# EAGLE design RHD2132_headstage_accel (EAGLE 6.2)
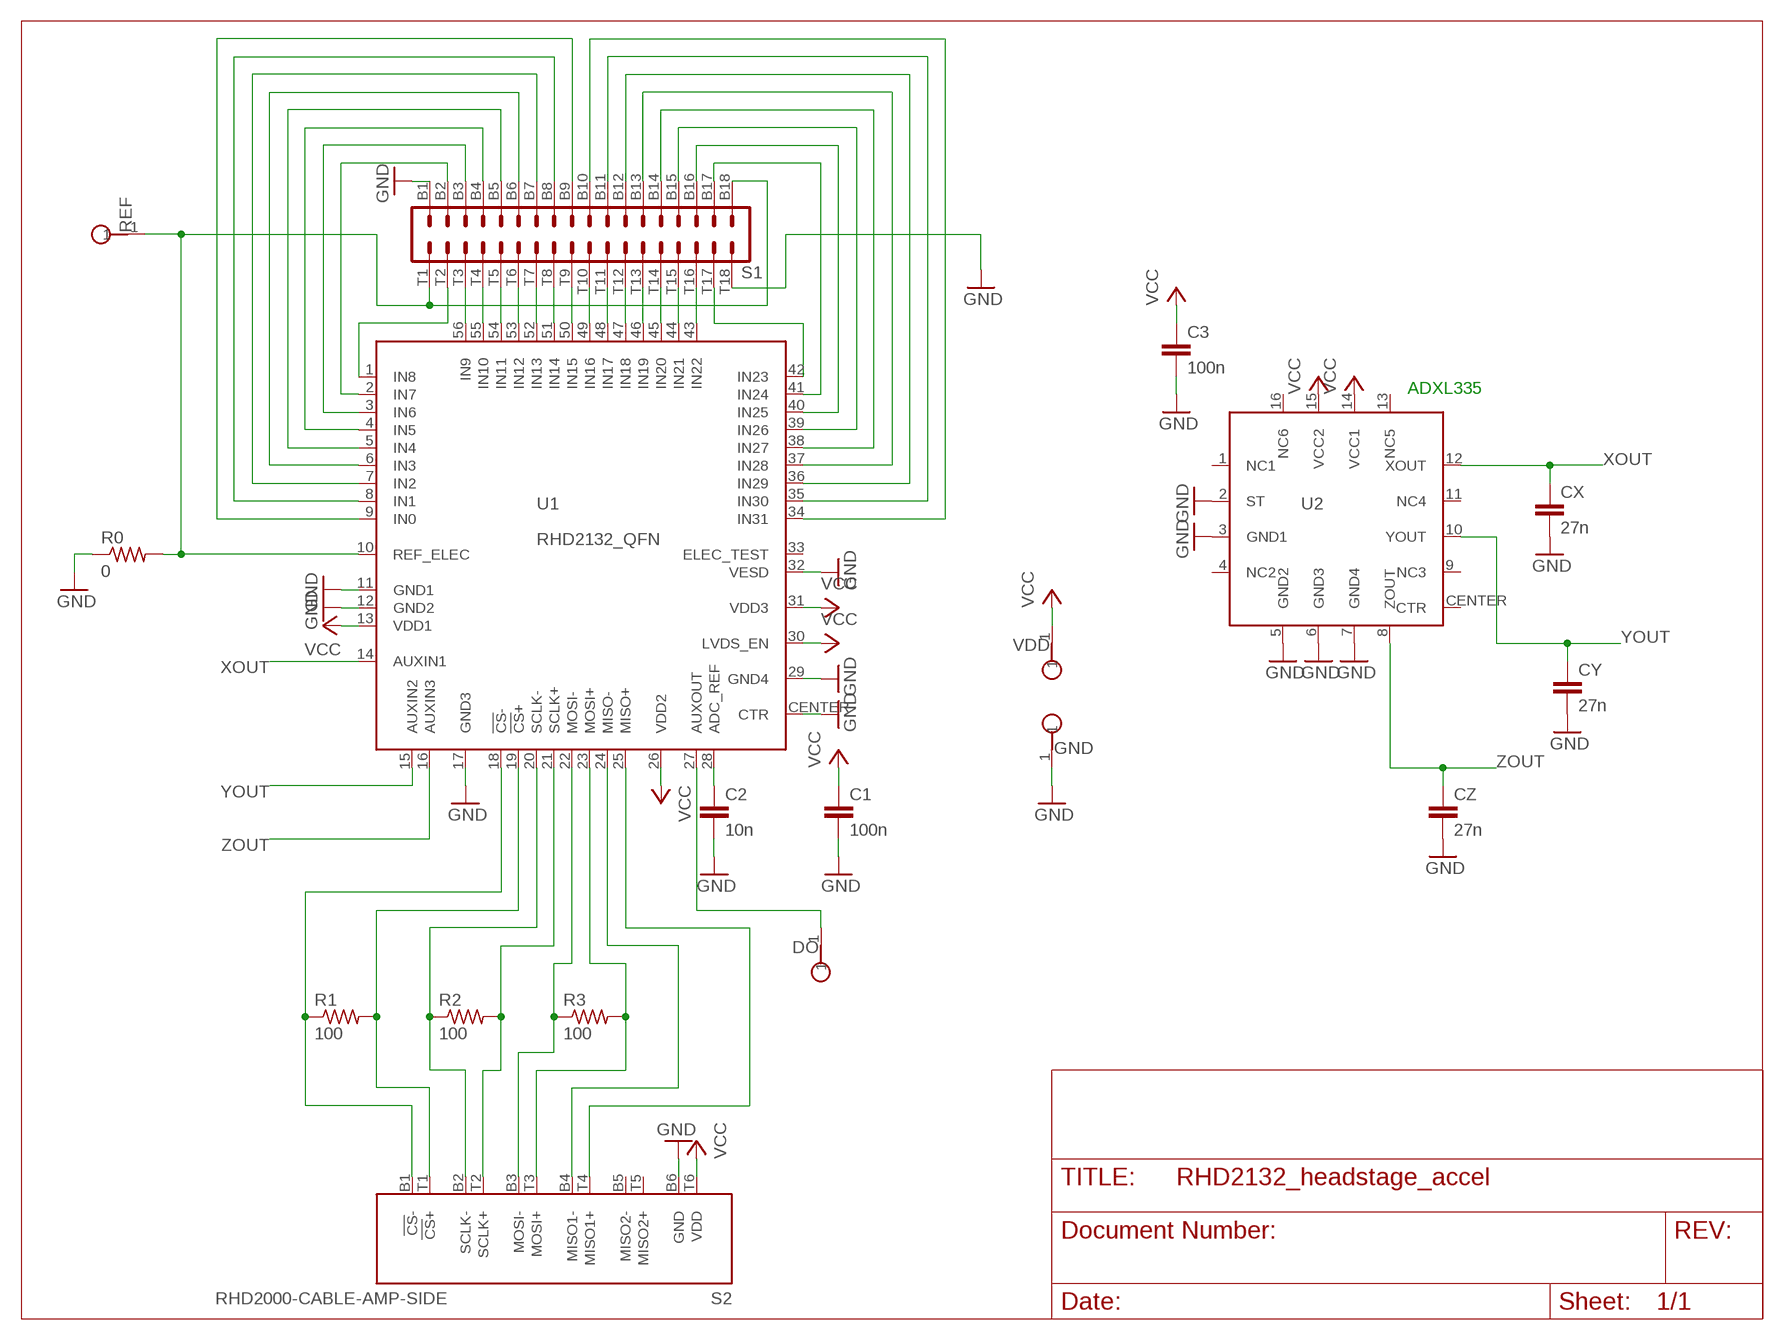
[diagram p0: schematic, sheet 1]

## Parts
C1  100n  C_0402  [0402]
C2  10n  C_0402  [0402]
C3  100n  C_0402  [0402]
CX  27n  C_0402  [0402]
CY  27n  C_0402  [0402]
CZ  27n  C_0402  [0402]
DO  TESTPOINT_SMALL  [TESTPOINT_SMALL]
GND  TESTPOINT_SMALL  [TESTPOINT_SMALL]
R0  0  R_0402  [0402]
R1  100  R_0402  [0402]
R2  100  R_0402  [0402]
R3  100  R_0402  [0402]
REF  TESTPOINT_SMALL  [TESTPOINT_SMALL]
S1  OMNETICS_A79025  [OMNETICS_A79025]
S2  RHD2000-CABLE-AMP-SIDE  [OMNETICS_PZN-12-AA]
U1  RHD2132_QFN  [QFN56_8_X_8_LARGE]
U2  ADXL335  [ADXL335]
VDD  TESTPOINT_SMALL  [TESTPOINT_SMALL]

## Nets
GND: C1.2 C2.2 C3.2 CX.2 CY.2 CZ.2 GND.1 R0.1 S1.B1 S1.T18 S2.B6(GND) U1.11(GND1) U1.12(GND2) U1.17(GND3) U1.29(GND4) U1.32(VESD) U1.CENTER(CTR) U2.2(ST) U2.3(GND1) U2.5(GND2) U2.6(GND3) U2.7(GND4)
N$1: R0.2 REF.1 S1.B18 S1.T1 U1.10(REF_ELEC)
N$2: S1.B3 U1.3(IN6)
N$3: S1.B2 U1.2(IN7)
N$4: S1.B4 U1.4(IN5)
N$5: S1.B5 U1.5(IN4)
N$6: S1.B6 U1.6(IN3)
N$7: S1.B7 U1.7(IN2)
N$8: S1.B8 U1.8(IN1)
N$9: S1.B9 U1.9(IN0)
N$10: S1.B10 U1.34(IN31)
N$11: R1.1 S2.B1(!CS!-) U1.18(!CS!-)
N$12: S1.B17 U1.41(IN24)
N$13: S1.B16 U1.40(IN25)
N$14: S1.B15 U1.39(IN26)
N$15: S1.B14 U1.38(IN27)
N$16: S1.B13 U1.37(IN28)
N$17: S1.B12 U1.36(IN29)
N$18: S1.B11 U1.35(IN30)
N$19: S1.T9 U1.50(IN15)
N$20: S1.T8 U1.51(IN14)
N$21: S1.T7 U1.52(IN13)
N$22: S1.T3 U1.56(IN9)
N$23: S1.T4 U1.55(IN10)
N$24: S1.T5 U1.54(IN11)
N$25: S1.T6 U1.53(IN12)
N$26: S1.T10 U1.49(IN16)
N$27: S1.T11 U1.48(IN17)
N$28: S1.T12 U1.47(IN18)
N$29: S1.T13 U1.46(IN19)
N$30: S1.T14 U1.45(IN20)
N$31: S1.T15 U1.44(IN21)
N$32: S1.T16 U1.43(IN22)
N$33: S1.T2 U1.1(IN8)
N$34: S1.T17 U1.42(IN23)
N$35: R1.2 S2.T1(!CS!+) U1.19(!CS!+)
N$36: R2.1 S2.B2(SCLK-) U1.20(SCLK-)
N$37: R2.2 S2.T2(SCLK+) U1.21(SCLK+)
N$38: R3.1 S2.B3(MOSI-) U1.22(MOSI-)
N$39: R3.2 S2.T3(MOSI+) U1.23(MOSI+)
N$40: S2.B4(MISO1-) U1.24(MISO-)
N$41: S2.T4(MISO1+) U1.25(MISO+)
N$42: C2.1 U1.28(ADC_REF)
N$43: DO.1 U1.27(AUXOUT)
VCC: C1.1 C3.1 S2.T6(VDD) U1.13(VDD1) U1.26(VDD2) U1.30(LVDS_EN) U1.31(VDD3) U2.14(VCC1) U2.15(VCC2) VDD.1
XOUT: CX.1 U1.14(AUXIN1) U2.12(XOUT)
YOUT: CY.1 U1.15(AUXIN2) U2.10(YOUT)
ZOUT: CZ.1 U1.16(AUXIN3) U2.8(ZOUT)
Unconnected: S2.B5(MISO2-) S2.T5(MISO2+) U1.33(ELEC_TEST) U2.1(NC1) U2.4(NC2) U2.9(NC3) U2.11(NC4) U2.13(NC5) U2.16(NC6) U2.CENTER(CTR)

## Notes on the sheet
- ADXL335

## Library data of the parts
C1-C3 CX CY CZ = RHD2000_eval_board:C: Capacitor
DO GND REF VDD = RHD2000_eval_board:TESTPOINT: PCB Test Point
R0 R1-R3 = RHD2000_eval_board:R: Resistor
S1 = RHD2000:OMNETICS_A79025
S2 = RHD2000:RHD2000-CABLE-AMP-SIDE
U1 = RHD2000:RHD2132
U2 = harrison:ADXL335

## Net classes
1 thick: width 1.016 mm
2 power: width 0.61 mm

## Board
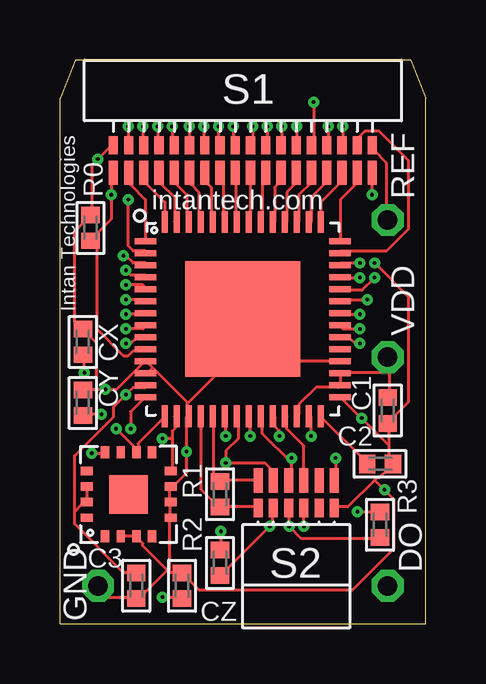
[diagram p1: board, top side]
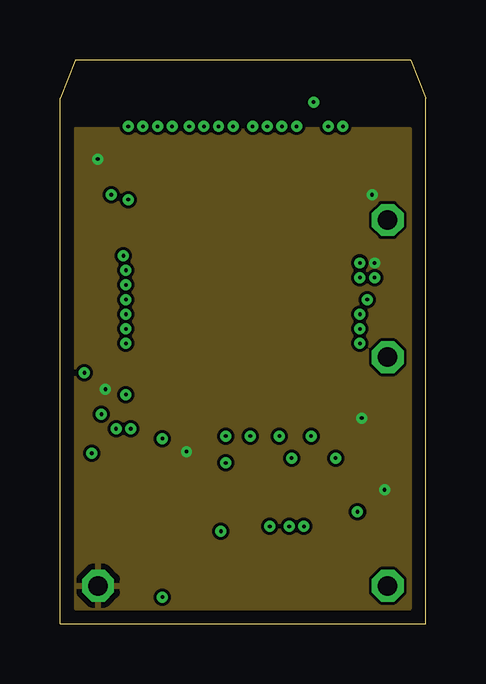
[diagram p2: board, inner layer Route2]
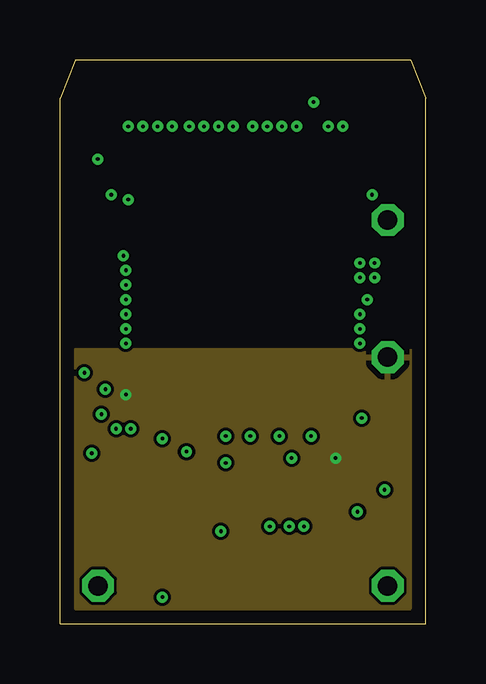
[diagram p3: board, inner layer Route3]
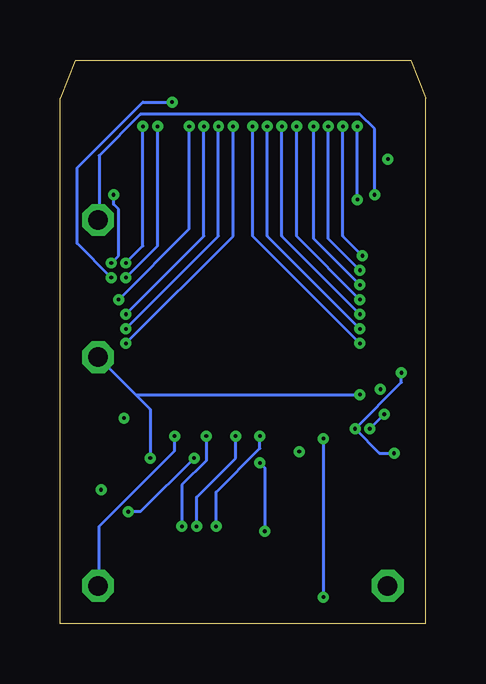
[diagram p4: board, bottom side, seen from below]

Size 15.24 x 23.5 mm. Coordinates in mm from the lower left corner, seen from the top.
Outline: 0,0 0,21.91 0.64,23.5 14.61,23.5 15.24,21.91 15.24,0 0,0
Copper layers (1*2+3*16): Top 0.035mm / dielectric 1.5mm / Route2 0.035mm / dielectric 0.15mm / Route3 0.035mm / dielectric 0.2mm / Bottom 0.035mm
Design rules: minimum track width 5mil, minimum drill 6mil, track to track 5mil, track to pad 5mil, pad to pad 5mil, via to via 5mil, smd to smd 5mil, copper to edge 15mil, drill to drill 15mil, minimum pad ring 10mil, minimum via ring 6mil, stop-mask expansion 4mil, vias tented up to drill 0mil, thermal gap 10mil

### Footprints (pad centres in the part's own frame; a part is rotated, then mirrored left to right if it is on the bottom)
0402 = smd 0.686 x 0.762: 1 -0.533,0; 2 0.533,0
TESTPOINT_SMALL = drill 0.813 octagon: 1 0,0
OMNETICS_A79025 = smd 0.381 x 0.762: B1 -5.397,-1.016; B2 -4.763,-1.016; B3 -4.128,-1.016; B4 -3.493,-1.016; B5 -2.857,-1.016; B6 -2.223,-1.016; B7 -1.587,-1.016; B8 -0.953,-1.016; B9 -0.318,-1.016; B10 0.318,-1.016; B11 0.953,-1.016; B12 1.587,-1.016; B13 2.223,-1.016; B14 2.857,-1.016; B15 3.493,-1.016; B16 4.128,-1.016; B17 4.763,-1.016; B18 5.397,-1.016 | smd 0.381 x 1.016: T1 -5.397,-2.159; T2 -4.763,-2.159; T3 -4.128,-2.159; T4 -3.493,-2.159; T5 -2.857,-2.159; T6 -2.223,-2.159; T7 -1.587,-2.159; T8 -0.953,-2.159; T9 -0.318,-2.159; T10 0.318,-2.159; T11 0.953,-2.159; T12 1.587,-2.159; T13 2.223,-2.159; T14 2.857,-2.159; T15 3.493,-2.159; T16 4.128,-2.159; T17 4.763,-2.159; T18 5.397,-2.159
OMNETICS_PZN-12-AA = smd 0.381 x 0.762: B1 1.587,-1.016; B2 0.953,-1.016; B3 0.318,-1.016; B4 -0.318,-1.016; B5 -0.953,-1.016; B6 -1.587,-1.016 | smd 0.381 x 1.016: T1 1.587,-2.159; T2 0.953,-2.159; T3 0.318,-2.159; T4 -0.318,-2.159; T5 -0.953,-2.159; T6 -1.587,-2.159
QFN56_8_X_8_LARGE = smd 0.9 x 0.25: 1 -4.05,3.25; 2 -4.05,2.75; 3 -4.05,2.25; 4 -4.05,1.75; 5 -4.05,1.25; 6 -4.05,0.75; 7 -4.05,0.25; 8 -4.05,-0.25; 9 -4.05,-0.75; 10 -4.05,-1.25; 11 -4.05,-1.75; 12 -4.05,-2.25; 13 -4.05,-2.75; 14 -4.05,-3.25; 29 4.05,-3.25; 30 4.05,-2.75; 31 4.05,-2.25; 32 4.05,-1.75; 33 4.05,-1.25; 34 4.05,-0.75; 35 4.05,-0.25; 36 4.05,0.25; 37 4.05,0.75; 38 4.05,1.25; 39 4.05,1.75; 40 4.05,2.25; 41 4.05,2.75; 42 4.05,3.25 | smd 0.25 x 0.9: 15 -3.25,-4.05; 16 -2.75,-4.05; 17 -2.25,-4.05; 18 -1.75,-4.05; 19 -1.25,-4.05; 20 -0.75,-4.05; 21 -0.25,-4.05; 22 0.25,-4.05; 23 0.75,-4.05; 24 1.25,-4.05; 25 1.75,-4.05; 26 2.25,-4.05; 27 2.75,-4.05; 28 3.25,-4.05; 43 3.25,4.05; 44 2.75,4.05; 45 2.25,4.05; 46 1.75,4.05; 47 1.25,4.05; 48 0.75,4.05; 49 0.25,4.05; 50 -0.25,4.05; 51 -0.75,4.05; 52 -1.25,4.05; 53 -1.75,4.05; 54 -2.25,4.05; 55 -2.75,4.05; 56 -3.25,4.05 | smd 4.8 x 4.8: CENTER 0,0
ADXL335 = smd 0.5 x 0.35: 1 -1.75,0.975; 2 -1.75,0.325; 3 -1.75,-0.325; 4 -1.75,-0.975; 9 1.75,-0.975; 10 1.75,-0.325; 11 1.75,0.325; 12 1.75,0.975 | smd 0.35 x 0.5: 5 -0.975,-1.75; 6 -0.325,-1.75; 7 0.325,-1.75; 8 0.975,-1.75; 13 0.975,1.75; 14 0.325,1.75; 15 -0.325,1.75; 16 -0.975,1.75 | smd 1.6 x 1.6: CENTER 0,0

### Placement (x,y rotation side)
C1  13.65,8.89 270 top
C2  13.34,6.67 0 top
C3  3.17,1.59 270 top
CX  0.95,11.75 90 top
CY  0.95,9.21 90 top
CZ  5.08,1.59 90 top
DO  13.65,1.59 0 top
GND  1.59,1.59 0 top
R0  1.27,16.5 270 top
R1  6.67,5.4 90 top
R2  6.67,2.54 90 top
R3  13.34,4.13 90 top
REF  13.65,16.83 90 top
S1  7.62,20.95 0 top
S2  9.84,3.81 180 top
U1  7.62,12.7 0 top
U2  2.86,5.4 90 top
VDD  13.65,11.11 0 top

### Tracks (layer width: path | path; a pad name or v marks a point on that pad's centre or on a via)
GND  (via drill 0.15)
  Top 0.127: 8.23,12.09 9.35,10.97 11.58,10.97 U1.32 | S1.B1 2.13,19.91 1.32,19.1 1.32,17.07 R0.1 1.22,16.97 0.61,16.36 0.61,12.6 0.91,12.29 CX.2 1.02,12.19 1.52,11.68 1.52,9.75 | 1.52,9.75 2.34,9.75 3.56,10.97 U1.11 3.66,10.87 3.86,10.67 | 1.52,9.75 1.02,9.75 CY.2 | 5.28,9.14 5.28,9.25 3.86,10.67 | 5.28,9.14 5.28,8.74 U1.17 5.28,8.64 5.28,6.3 4.67,5.69 U2.7 4.57,5.69 4.57,5.08 U2.6 4.57,4.98 4.57,4.47 U2.5 4.57,4.37 4.57,2.13 | 3.86,10.67 3.66,10.46 U1.12 | 5.28,9.14 8.23,12.09 | 8.23,12.09 U1.CENTER | 13.11,5.99 13.21,6.1 13.31,6.1 13.72,6.5 | 13.11,5.99 11.99,4.88 11.48,4.88 S2.B6 | 13.72,6.5 13.82,6.6 C2.2 13.72,6.5 | 13.72,6.5 13.72,7.42 | 13.72,7.42 13.72,8.33 C1.2 13.72,8.43 14.53,9.25 14.53,13.61 v13.11,15.04 | 13.72,7.42 11.68,9.45 U1.29 | U2.2 3.15,3.66 U2.3 3.25,3.56 3.45,3.35 3.45,3.25 4.47,2.23 | 4.57,2.13 4.47,2.23 | 5.08,2.13 4.57,2.13 | GND.1 1.63,1.52 2.03,1.12 3.15,1.12 C3.2 3.25,1.02 4.47,2.23 | 13.11,5.99 13.92,5.18 13.92,3.15 12.19,1.42 5.79,1.42 5.08,2.13 | 5.08,2.13 CZ.2 | v13.01,17.88 13.01,18.8 S1.T18
  Bottom 0.127: v13.01,17.88 13.01,17.48 12.8,17.27 12.8,15.34 v13.11,15.04
  other vias: 12.57,8.57 13.53,5.59 5.27,7.18 1.57,19.37 1.89,9.78
  pour Route2: 0.64,0.64 14.61,0.64 14.61,20.64 0.64,20.64
N$1  (via drill 0.15)
  Top 0.127: S1.B18 13.11,19.91 13.11,19.71 13.61,19.2 13.61,16.87 REF.1 | 1.52,16.26 2.13,16.87 v2.13,17.88 2.13,18.8 S1.T1 | 1.52,16.26 1.32,16.05 R0.2 1.52,16.26 | 1.52,16.26 1.52,12.29 2.64,11.18 2.85,11.18 3.05,11.38 3.56,11.38 U1.10
  Bottom 0.127: v2.13,17.88 2.13,20.62 2.74,21.23 11.89,21.23 13.61,19.51 13.61,16.87 REF.1
N$2  (via drill 0.15)
  Top 0.127: v3.45,20.73 3.45,20.02 S1.B3 | v2.64,15.34 2.74,15.34 3.05,15.04 3.56,15.04 U1.3
  Bottom 0.127: v3.45,20.73 3.45,16.15 v2.64,15.34
N$3  (via drill 0.15)
  Top 0.127: v2.85,20.73 2.85,20.02 S1.B2 | v2.85,17.68 2.85,15.75 3.05,15.54 3.56,15.54 U1.2
  Bottom 0.127: v2.85,17.68 v2.85,20.73
N$4  (via drill 0.15)
  Top 0.127: v4.06,20.73 4.06,20.02 S1.B4 | v2.74,14.73 2.95,14.53 3.56,14.53 U1.4
  Bottom 0.127: v4.06,20.73 4.06,16.05 v2.74,14.73
N$5  (via drill 0.15)
  Top 0.127: v4.67,20.73 4.67,20.02 S1.B5 | v2.74,14.12 3.45,14.12 3.56,14.02 U1.5
  Bottom 0.127: v4.67,20.73 4.67,16.05 v2.74,14.12
N$6  (via drill 0.15)
  Top 0.127: v5.38,20.73 5.38,20.02 S1.B6 | v2.74,13.51 3.56,13.51 U1.6
  Bottom 0.127: v5.38,20.73 5.38,16.15 v2.74,13.51
N$7  (via drill 0.15)
  Top 0.127: v5.99,20.73 5.99,20.02 S1.B7 | v2.74,12.9 3.56,12.9 U1.7
  Bottom 0.127: v5.99,20.73 5.99,16.15 v2.74,12.9
N$8  (via drill 0.15)
  Top 0.127: v6.6,20.73 6.6,20.02 S1.B8 | v2.74,12.29 3.45,12.29 3.56,12.39 U1.8
  Bottom 0.127: v6.6,20.73 6.6,16.15 v2.74,12.29
N$9  (via drill 0.15)
  Top 0.127: v7.21,20.73 7.21,20.02 S1.B9 | v2.74,11.68 2.95,11.68 3.15,11.89 3.56,11.89 U1.9
  Bottom 0.127: v7.21,20.73 7.21,16.15 v2.74,11.68
N$10  (via drill 0.15)
  Top 0.127: v8.03,20.73 8.03,20.02 S1.B10 | v12.5,11.68 12.29,11.68 12.09,11.89 11.68,11.89 U1.34
  Bottom 0.127: v8.03,20.73 8.03,16.15 v12.5,11.68
N$11
  Top 0.127: S2.B1 8.23,4.88 6.71,4.88 R1.1 6.6,4.88 5.89,5.59 5.89,8.64 U1.18
N$12
  Top 0.127: S1.B17 12.39,20.02 12.39,20.22 12.7,20.52 13.31,20.52 14.53,19.3 14.53,16.46 13.61,15.54 11.68,15.54 U1.41
N$13  (via drill 0.15)
  Top 0.127: v11.79,20.73 11.79,20.02 S1.B16 | v12.5,15.04 11.68,15.04 U1.40
  Bottom 0.127: v11.79,20.73 11.79,15.75 v12.5,15.04
N$14  (via drill 0.15)
  Top 0.127: v11.18,20.73 11.18,20.02 S1.B15 | v12.5,14.43 11.68,14.43 U1.39
  Bottom 0.127: v11.18,20.73 11.18,15.75 v12.5,14.43
N$15  (via drill 0.15)
  Top 0.127: v10.57,21.74 10.57,20.02 S1.B14 | v13.11,14.43 12.6,13.92 11.68,13.92 U1.38
  Bottom 0.127: v10.57,21.74 11.79,21.74 14.53,19 14.53,15.85 v13.11,14.43
N$16  (via drill 0.15)
  Top 0.127: v9.86,20.73 9.86,20.02 S1.B13 | v12.8,13.51 11.68,13.51 U1.37
  Bottom 0.127: v9.86,20.73 9.86,16.46 v12.8,13.51
N$17  (via drill 0.15)
  Top 0.127: v9.25,20.73 9.25,20.02 S1.B12 | v12.5,12.9 11.68,12.9 U1.36
  Bottom 0.127: v9.25,20.73 9.25,16.15 v12.5,12.9
N$18  (via drill 0.15)
  Top 0.127: v8.64,20.73 8.64,20.02 S1.B11 | v12.5,12.29 11.79,12.29 11.68,12.39 U1.35
  Bottom 0.127: v8.64,20.73 8.64,16.15 v12.5,12.29
N$19
  Top 0.127: U1.50 7.32,16.76 7.32,18.8 S1.T9
N$20
  Top 0.127: U1.51 6.81,16.76 6.81,18.69 6.71,18.8 S1.T8
N$21
  Top 0.127: U1.52 6.3,16.76 6.3,18.19 6.1,18.39 6.1,18.8 S1.T7
N$22
  Top 0.127: U1.56 4.37,16.76 4.37,17.58 3.56,18.39 3.56,18.8 S1.T3
N$23
  Top 0.127: U1.55 4.78,16.76 4.78,17.78 4.17,18.39 4.17,18.8 S1.T4
N$24
  Top 0.127: U1.54 5.28,16.76 5.28,17.88 4.78,18.39 4.78,18.8 S1.T5
N$25
  Top 0.127: U1.53 5.79,16.76 5.79,17.98 5.49,18.29 5.49,18.8 S1.T6
N$26
  Top 0.127: U1.49 7.92,16.76 7.92,18.8 S1.T10
N$27
  Top 0.127: U1.48 8.43,16.76 8.43,18.69 8.53,18.8 S1.T11
N$28
  Top 0.127: U1.47 8.94,16.76 8.94,18.19 9.14,18.39 9.14,18.8 S1.T12
N$29
  Top 0.127: U1.46 9.45,16.76 9.45,17.98 9.75,18.29 9.75,18.8 S1.T13
N$30
  Top 0.127: U1.45 9.96,16.76 9.96,17.88 10.46,18.39 10.46,18.8 S1.T14
N$31
  Top 0.127: U1.44 10.46,16.76 10.46,17.78 11.07,18.39 11.07,18.8 S1.T15
N$32
  Top 0.127: U1.43 10.87,16.76 10.87,17.58 11.68,18.39 11.68,18.8 S1.T16
N$33
  Top 0.127: U1.1 3.56,15.95 3.56,17.68 2.95,18.29 2.95,18.8 S1.T2
N$34
  Top 0.127: U1.42 11.68,15.95 11.68,17.68 12.29,18.29 12.29,18.8 S1.T17
N$35
  Top 0.127: S2.T1 8.23,5.99 6.71,5.99 R1.2 6.4,6.2 6.4,8.64 U1.19
N$36  (via drill 0.15)
  Top 0.127: R2.1 6.71,2.03 v8.74,4.06 8.84,4.17 8.84,4.78 S2.B2 | v6.91,7.82 6.91,8.64 U1.20
  Bottom 0.127: v6.91,7.82 6.91,7.32 8.74,5.49 v8.74,4.06
N$37  (via drill 0.15)
  Top 0.127: v6.71,3.86 6.71,3.15 R2.2 | U1.21 7.42,8.64 7.42,7.72 6.91,7.21 v6.91,6.71 8.53,6.71 8.84,6.4 8.84,5.99 S2.T2
  Bottom 0.127: v6.71,3.86 6.71,6.5 v6.91,6.71
N$38  (via drill 0.15)
  Top 0.127: S2.B3 9.55,4.78 v9.55,4.06 10.06,3.56 13.31,3.56 R3.1 | v7.92,7.82 7.92,8.64 U1.22
  Bottom 0.127: v7.92,7.82 7.92,6.91 9.55,5.28 v9.55,4.06
N$39  (via drill 0.15)
  Top 0.127: v12.39,4.67 13.31,4.67 R3.2 | 9.65,6.71 9.65,6.1 S2.T3 | 9.65,6.71 8.43,7.92 8.43,8.64 U1.23 | 9.65,6.71 v9.65,6.91
  Bottom 0.127: v12.39,4.67 11.89,4.67 v9.65,6.91
N$40  (via drill 0.15)
  Top 0.127: v10.16,4.06 S2.B4 | v9.14,7.82 9.14,8.03 8.94,8.23 8.94,8.64 U1.24
  Bottom 0.127: v10.16,4.06 10.16,5.79 9.14,6.81 v9.14,7.82
N$41
  Top 0.127: S2.T4 10.16,7.42 9.45,8.13 9.45,8.64 U1.25
N$42
  Top 0.127: C2.1 12.8,6.71 10.87,8.64 U1.28
N$43  (via drill 0.15)
  Top 0.127: v10.46,7.82 10.46,8.64 U1.27
  Bottom 0.127: v10.46,7.82 10.46,7.21 13.61,4.06 13.61,1.63 DO.1
VCC  (via drill 0.15)
  Top 0.127: U2.14 1.12,5.69 U2.15 1.02,4.98 0.91,4.98 0.61,4.67 | 0.61,4.67 0.61,4.17 2.64,2.13 3.15,2.13 C3.1 | 0.61,4.67 0.61,7.01 2.23,8.64 2.23,9.04 v2.74,9.55 3.05,9.86 3.56,9.86 U1.13 | U1.26 9.96,8.74 9.96,9.14 10.67,9.86 11.58,9.86 U1.30 11.68,9.96 11.68,10.36 U1.31 11.68,10.46 13.72,10.46 | 13.72,10.46 13.72,11.07 VDD.1 13.72,10.46 | 13.72,10.46 13.72,9.45 C1.1 | v11.48,6.91 11.48,5.99 S2.T6
  Bottom 0.127: v11.48,6.91 11.48,8.94 12.09,9.55 | VDD.1 12.09,9.55 | 12.09,9.55 v2.74,9.55
  pour Route3: 0.64,0.64 14.61,0.64 14.61,11.43 0.64,11.43
XOUT  (via drill 0.15)
  Top 0.127: v1.32,7.11 1.83,7.11 U2.12 | v2.95,8.13 2.95,8.84 3.56,9.45 U1.14 | v1.02,10.46 1.02,11.18 CX.1
  Bottom 0.127: v1.32,7.11 1.93,7.11 v2.95,8.13 1.02,10.06 v1.02,10.46
YOUT  (via drill 0.15)
  Top 0.127: 3.25,7.21 3.25,7.52 4.37,8.64 U1.15 | v1.73,8.74 1.02,8.74 CY.1 | 3.25,7.21 v2.34,8.13 | 3.25,7.21 U2.10
  Bottom 0.127: v2.34,8.13 v1.73,8.74
ZOUT  (via drill 0.15)
  Top 0.127: 4.67,7.72 4.67,8.03 4.78,8.13 4.78,8.64 U1.16 | 4.67,7.72 4.67,6.4 U2.8 | v4.27,1.12 5.08,1.12 CZ.1 | 4.67,7.72 v4.27,7.72
  Bottom 0.127: v4.27,7.72 v4.27,1.12

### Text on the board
tPlace: intantech.com | Intan Technologies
